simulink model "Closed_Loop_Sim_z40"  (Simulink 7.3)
settings: Solver=ode4  StartTime=0.0  StopTime=40  FixedStep=0.04  RelTol=1e-3
InitFcn:
  | d2r=pi/180; r2d=180/pi;
  | [Av1, Bv1, Cv1, Dv1]= plant_flxcont;              % Continuous Plant
  | [Av4, Bv4, Cv4, Dv4]= plant_flxz40ms;             % Discrete Plant at 40 msec
  | [Acz, Bcz, Ccz, Dcz]= controller_z;               % Discrete Stage-2 Controller (T=0.04)
  | [Acs, Bcs, Ccs, Dcs]= controller_s;               % Continuous Stage-2 Controller (T=0)
StartFcn:
  | d2r=pi/180; r2d=180/pi;
  | [Av1, Bv1, Cv1, Dv1]= plant_flxcont;              % Continuous Plant
  | [Av4, Bv4, Cv4, Dv4]= plant_flxz40ms;             % Discrete Plant at 40 msec
  | [Acz, Bcz, Ccz, Dcz]= controller_z;               % Discrete Stage-2 Controller (T=0.04)
  | [Acs, Bcs, Ccs, Dcs]= controller_s;               % Continuous Stage-2 Controller (T=0)
StopFcn:
  | Pl
undefined symbols (not defined in the file or in its folder): Acz, Av4, Bcz, Bv4, Ccz, Cv4, Dcz, Dv4

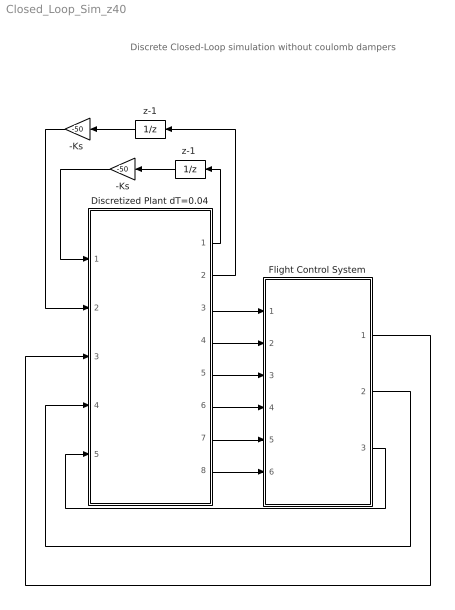
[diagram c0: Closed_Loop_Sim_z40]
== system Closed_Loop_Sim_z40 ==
  note: Discrete Closed-Loop simulation without coulomb dampers
  -Ks : Gain  Gain=-50  ParameterDataType=sfix(16)  ParameterScaling=2^0  OutDataType=sfix(16)  OutScaling=2^0
  "-Ks " : Gain  Gain=-50  ParameterDataType=sfix(16)  ParameterScaling=2^0  OutDataType=sfix(16)  OutScaling=2^0
  Discretized Plant dT=0.04 : Subsystem
  Flight Control System : Subsystem
  z-1 : UnitDelay  SampleTime=0.04
  "z-1 " : UnitDelay  SampleTime=0.04
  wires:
  Discretized Plant dT=0.04/3(phi) -> Flight Control System/1(Phi)
  Discretized Plant dT=0.04/4(theta) -> Flight Control System/2(Theta)
  Discretized Plant dT=0.04/5(psi) -> Flight Control System/3(Psi)
  Discretized Plant dT=0.04/6(P) -> Flight Control System/4(P)
  Discretized Plant dT=0.04/7(Q) -> Flight Control System/5(Q)
  Discretized Plant dT=0.04/8(R) -> Flight Control System/6(R)
  Flight Control System/1(DP-TVC) -> Discretized Plant dT=0.04/3(DP)
  Flight Control System/2(DQ-TVC) -> Discretized Plant dT=0.04/4(DQ)
  Flight Control System/3(DR-TVC) -> Discretized Plant dT=0.04/5(DR)
  "-Ks "/1 -> Discretized Plant dT=0.04/2(F-right)
  -Ks/1 -> Discretized Plant dT=0.04/1(F-left)
  Discretized Plant dT=0.04/1(dZ-Left) -> "z-1 "/1
  Discretized Plant dT=0.04/2(dZ-Rght) -> z-1/1
  z-1/1 -> "-Ks "/1
  "z-1 "/1 -> -Ks/1

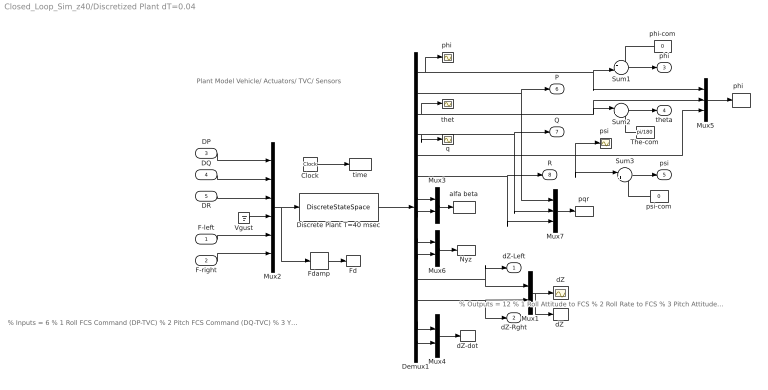
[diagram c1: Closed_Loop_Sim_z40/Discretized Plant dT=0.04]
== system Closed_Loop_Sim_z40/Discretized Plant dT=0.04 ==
  note: Plant Model Vehicle/ Actuators/ TVC/ Sensors
  note: % Inputs = 6 % 1 Roll FCS Command (DP-TVC) % 2 Pitch FCS Command (DQ-TVC) % 3 Yaw FCS Command (DR-TVC) % 4 Wind-Gust Velocity (ft/sec) % 5 Left Coulomb Damper Force % 6 Right Coulomb Damper Force
  note: % Outputs = 12 % 1 Roll Attitude to FCS % 2 Roll Rate to FCS % 3 Pitch Attitude to FCS % 4 Pitch Rate to FCS % 5 Yaw Attitude to FCS % 6 Yaw Rate to FCS % 7 Angle of Attack, alpha (rad) % 8 Angle of Sideslip, beta (rad) % 9 Normal Accelerometer, Nz (ft/sec^2) % 10 Lateral Accelerometer, Ny (ft/sec^2) % 11 Left Damper Extension (ft) % 12 Right Damper Extension (ft) % 13 Left Damper Rate (ft/sec) % 14 Right Damper Rate (ft/s)
  F-left : Inport  OutDataType=sfix(16)  OutScaling=2^0
  F-right : Inport  Port=2  OutDataType=sfix(16)  OutScaling=2^0
  DP : Inport  Port=3  OutDataType=sfix(16)  OutScaling=2^0
  DQ : Inport  Port=4  OutDataType=sfix(16)  OutScaling=2^0
  DR : Inport  Port=5  OutDataType=sfix(16)  OutScaling=2^0
  Clock : Clock
  Demux1 : Demux  Outputs=14
  Discrete Plant T=40 msec : DiscreteStateSpace  A=Av4  B=Bv4  C=Cv4  D=Dv4  SampleTime=0.04
  Fd : ToWorkspace  VariableName=Fd  SampleTime=-1  SaveFormat=Array
  Fdamp : Selector  InputPortWidth=6  IndexOptions=Index vector (dialog)  Indices="[5  6]"  OutputSizes=1
  Mux{1,3..4,6} (4 alike) : Mux  Inputs=2
  Mux2 : Mux  Inputs=6
  Mux5 : Mux  Inputs=3
  Mux7 : Mux  Inputs=3
  Nyz : ToWorkspace  VariableName=Nyz  SampleTime=-1  SaveFormat=Array
  Sum1 : Sum  Inputs=-+|  OutDataType=sfix(16)  OutScaling=2^0
  Sum2 : Sum  Inputs=|+-  OutDataType=sfix(16)  OutScaling=2^0
  Sum3 : Sum  Inputs=|+-  OutDataType=sfix(16)  OutScaling=2^0
  The-com : Constant  Value=pi/180  OutDataType=sfix(16)  OutScaling=2^0
  Vgust : Ground
  alfa beta : ToWorkspace  VariableName=albet  SampleTime=-1  SaveFormat=Array
  dZ : Scope
  "dZ " : ToWorkspace  VariableName=dZ  SampleTime=-1  SaveFormat=Array
  dZ-dot : ToWorkspace  VariableName=dZd  SampleTime=-1  SaveFormat=Array
  "phi " : Scope
  "phi   " : ToWorkspace  VariableName=attit  SampleTime=-1  SaveFormat=Array
  phi-com : Constant  Value=0  OutDataType=sfix(16)  OutScaling=2^0
  pqr : ToWorkspace  VariableName=pqr  SampleTime=-1  SaveFormat=Array
  "psi " : Scope
  psi-com : Constant  Value=0  OutDataType=sfix(16)  OutScaling=2^0
  q : Scope
  thet : Scope
  time : ToWorkspace  VariableName=time  SampleTime=-1  SaveFormat=Array
  dZ-Left : Outport  OutDataType=sfix(16)  OutScaling=2^0
  dZ-Rght : Outport  Port=2  OutDataType=sfix(16)  OutScaling=2^0
  phi : Outport  Port=3  OutDataType=sfix(16)  OutScaling=2^0
  theta : Outport  Port=4  OutDataType=sfix(16)  OutScaling=2^0
  psi : Outport  Port=5  OutDataType=sfix(16)  OutScaling=2^0
  P : Outport  Port=6  OutDataType=sfix(16)  OutScaling=2^0
  Q : Outport  Port=7  OutDataType=sfix(16)  OutScaling=2^0
  R : Outport  Port=8  OutDataType=sfix(16)  OutScaling=2^0
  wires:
  F-left/1 -> Mux2/5
  F-right/1 -> Mux2/6
  DP/1 -> Mux2/1
  DQ/1 -> Mux2/2
  DR/1 -> Mux2/3
  Demux1/7 -> Mux3/1
  Demux1/9 -> Mux6/1
  Demux1/11 -> Mux1/1, dZ-Left/1
  Demux1/12 -> Mux1/2, dZ-Rght/1
  Mux2/1 -> Discrete Plant T=40 msec/1, Fdamp/1
  Mux3/1 -> alfa beta/1
  Mux6/1 -> Nyz/1
  Vgust/1 -> Mux2/4
  Demux1/2 -> P/1, Mux7/1
  Demux1/6 -> R/1, Mux7/3
  Discrete Plant T=40 msec/1 -> Demux1/1
  Mux1/1 -> dZ/1, "dZ "/1
  Sum2/1 -> theta/1
  Demux1/3 -> thet/1, Sum2/1, Mux5/2
  The-com/1 -> Sum2/2
  Demux1/1 -> "phi "/1, Sum1/2, Mux5/1
  Sum1/1 -> phi/1
  phi-com/1 -> Sum1/1
  Sum3/1 -> psi/1
  Demux1/5 -> Sum3/1, Mux5/3, "psi "/1
  psi-com/1 -> Sum3/2
  Demux1/4 -> q/1, Q/1, Mux7/2
  Fdamp/1 -> Fd/1
  Clock/1 -> time/1
  Demux1/13 -> Mux4/1
  Demux1/14 -> Mux4/2
  Mux4/1 -> dZ-dot/1
  Mux7/1 -> pqr/1
  Mux5/1 -> "phi   "/1
  Demux1/8 -> Mux3/2
  Demux1/10 -> Mux6/2

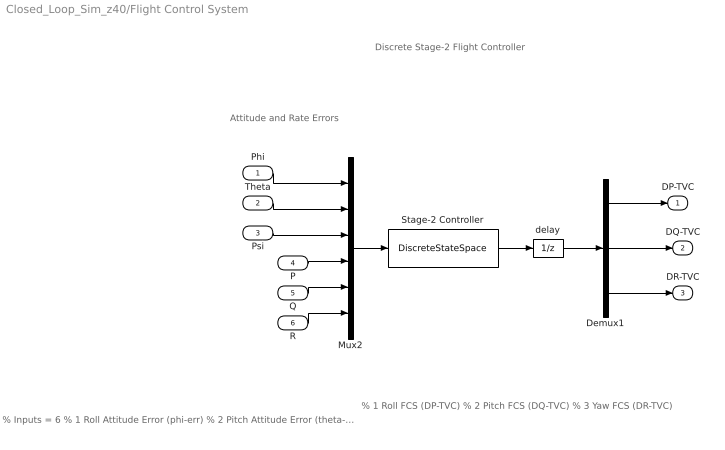
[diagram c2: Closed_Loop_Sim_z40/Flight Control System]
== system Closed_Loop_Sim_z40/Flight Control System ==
  note: Discrete Stage-2 Flight Controller
  note: Attitude and Rate Errors
  note: % Inputs = 6 % 1 Roll Attitude Error (phi-err) % 2 Pitch Attitude Error (theta-err) % 3 Yaw Attitude Error (psi-err) % 4 Roll Rate Error (p-err) % 5 Pitch Rate Error (q-err) % 6 Yaw Rate Error (r-err)
  note: % 1 Roll FCS (DP-TVC) % 2 Pitch FCS (DQ-TVC) % 3 Yaw FCS (DR-TVC)
  Phi : Inport  OutDataType=sfix(16)  OutScaling=2^0
  Theta : Inport  Port=2  OutDataType=sfix(16)  OutScaling=2^0
  Psi : Inport  Port=3  OutDataType=sfix(16)  OutScaling=2^0
  P : Inport  Port=4  OutDataType=sfix(16)  OutScaling=2^0
  Q : Inport  Port=5  OutDataType=sfix(16)  OutScaling=2^0
  R : Inport  Port=6  OutDataType=sfix(16)  OutScaling=2^0
  Demux1 : Demux  Outputs=3
  Mux2 : Mux  Inputs=6
  Stage-2 Controller : DiscreteStateSpace  A=Acz  B=Bcz  C=Ccz  D=Dcz  SampleTime=0.04
  delay : UnitDelay  SampleTime=0.04
  DP-TVC : Outport  OutDataType=sfix(16)  OutScaling=2^0
  DQ-TVC : Outport  Port=2  OutDataType=sfix(16)  OutScaling=2^0
  DR-TVC : Outport  Port=3  OutDataType=sfix(16)  OutScaling=2^0
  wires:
  Q/1 -> Mux2/5
  R/1 -> Mux2/6
  Phi/1 -> Mux2/1
  Theta/1 -> Mux2/2
  Psi/1 -> Mux2/3
  Mux2/1 -> Stage-2 Controller/1
  P/1 -> Mux2/4
  Demux1/2 -> DQ-TVC/1
  Demux1/1 -> DP-TVC/1
  Demux1/3 -> DR-TVC/1
  delay/1 -> Demux1/1
  Stage-2 Controller/1 -> delay/1
